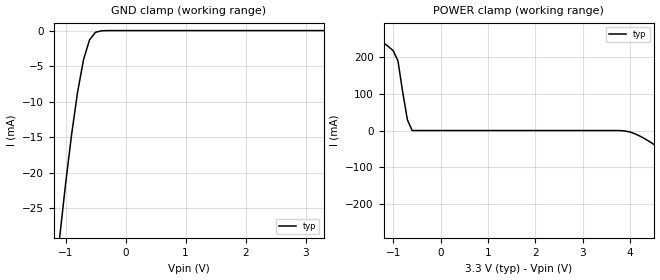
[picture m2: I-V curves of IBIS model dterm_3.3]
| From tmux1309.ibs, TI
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| dterm_3.3
[Model]   dterm_3.3
Model_type   Terminator
|   typ   min   max
C_comp   6.362683e-12   NA   NA
[Voltage Range]   3.3   NA   NA
[Temperature Range]   27   NA   NA
[Power Clamp Reference]   3.3   NA   NA
[GND Clamp Reference]   0   NA   NA
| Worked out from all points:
|   GND clamp passes 1 mA (typ) near -0.57 V on its own axis
|   POWER clamp passes 1 mA (typ) near -0.60 V on its own axis
[GND Clamp]
|   Voltage   I(typ)   I(min)   I(max)
-6.6V     -37.87kA   NA         NA
-1.1V     -29.29mA   NA         NA
-1V       -21.66mA   NA         NA
-900mV    -14.71mA   NA         NA
-800mV    -8.713mA   NA         NA
-700mV    -4.101mA   NA         NA
-600mV    -1.315mA   NA         NA
-500mV    -237.2uA   NA         NA
-400mV    -25.07uA   NA         NA
-300mV    -1.692uA   NA         NA
3.3V      810.6pA    NA         NA
[POWER Clamp]
|   Voltage   I(typ)   I(min)   I(max)
-3.3V     436.9mA    NA         NA
-1.7V     283.9mA    NA         NA
-1.1V     229.1mA    NA         NA
-1V       218mA      NA         NA
-900mV    190.3mA    NA         NA
-700mV    29.2mA     NA         NA
-600mV    58.4uA     NA         NA
4.1V      -8.713mA   NA         NA
4.9V      -73.61mA   NA         NA
6.2V      -208.8mA   NA         NA
6.3V      -289.2mA   NA         NA
6.6V      -1.138kA   NA         NA
